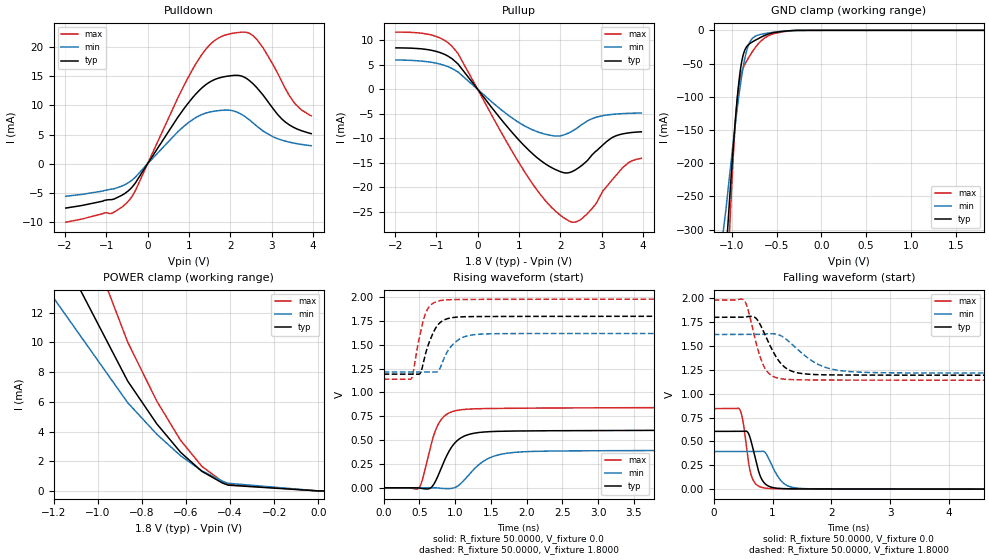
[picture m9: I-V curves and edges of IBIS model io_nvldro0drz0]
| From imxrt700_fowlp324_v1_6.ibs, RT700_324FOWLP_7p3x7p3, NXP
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[Model] io_nvldro0drz0
|   Model io_nvldro0drz0
| This model was characterised for following simulation conditions:
| External (pad) voltage:
|   - Typ: 1.8V,   - Min: 1.62V,   - Max: 1.98V
| Library cells for typ/min/max conditions are connected as defined below:
|  ipp_io - External Pad
|  ipp_do - Core Input
|  ipp_obe - Output Buffer Enable
|  config1v21v8 - gnde
|  drive0 - gnd
|  drive1 - gnd
|  gnd - gnd
|  gnde - gnde
|  ncgather - NC
|  vdd - vdd
|  vdde1v8 - vdde1v8
| All other pins connected to ground
Model_type I/O
Polarity   Non-Inverting
Enable   Active-Low
Vinl =   0.5400V
Vinh =   1.2600V
Vmeas =  0.9000V
Cref =   30.0000pF
Rref =   1.0000M
Vref =   1.8000V
C_comp   2.6144pF   2.5653pF   2.7096pF
|C_comp_pullup   1.3317pF   1.3902pF   1.2759pF
|C_comp_pulldown   0.0F   0.0F   0.0F
[Model Spec]
| variable   typ   min   max
Vinh   1.2600V   NA   NA
Vinl   0.5400V   NA   NA
Vref   1.8000V   1.8000V   1.8000V
Cref   30.0000pF   30.0000pF   30.0000pF
Rref   1.0000M   1.0000M   1.0000M
[Temperature Range]   25.0000   0.1250k   -40.0000
[Voltage Range]   1.8000V   1.6200V   1.9800V
[Pullup Reference]   1.8000V   1.6200V   1.9800V
[Pulldown Reference]   0.0V   0.0V   0.0V
[POWER Clamp Reference]   1.8000V   1.6200V   1.9800V
[GND Clamp Reference]   0.0V   0.0V   0.0V
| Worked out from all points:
|   slope of the pulldown table from 0 to 0.27 V, typ, clamps not added: 91.8 ohm
|   slope of the pullup table from 0 to 0.27 V, typ, clamps not added: 90.9 ohm
|   GND clamp passes 1 mA (typ) near -0.39 V on its own axis
|   POWER clamp passes 1 mA (typ) near -0.49 V on its own axis
|   rising waveform, R_fixture 50.0000, V_fixture 0.0: 20-80 % time 255ps typ, 362ps min, 198ps max; typ from 0 V to 0.605 V
|   rising waveform, R_fixture 50.0000, V_fixture 1.8000: 20-80 % time 173ps typ, 209ps min, 142ps max; typ from 1.19 V to 1.8 V
|   falling waveform, R_fixture 50.0000, V_fixture 0.0: 20-80 % time 159ps typ, 220ps min, 121ps max; typ from 0.605 V to 0 V
|   falling waveform, R_fixture 50.0000, V_fixture 1.8000: 20-80 % time 319ps typ, 521ps min, 225ps max; typ from 1.8 V to 1.19 V
[Pulldown]
|Voltage   I(typ)   I(min)   I(max)
-1.98V    -7.616mA   -5.589mA   -10.04mA
-876mV    -6.173mA   -4.375mA   -8.533mA
-468mV    -4.664mA   -3.281mA   -6.446mA
1.104V    11.45mA    7.63mA     16.37mA
1.464V    13.83mA    8.787mA    20.09mA
1.8V      14.84mA    9.158mA    21.85mA
2.232V    15.1mA     8.619mA    22.54mA
2.544V    13.77mA    7.047mA    22mA
2.796V    11.75mA    5.585mA    19.87mA
3.336V    7.128mA    3.861mA    12.86mA
3.624V    5.93mA     3.417mA    9.865mA
3.96V     5.157mA    3.077mA    8.199mA
[Pullup]
|Voltage   I(typ)   I(min)   I(max)
-1.98V    8.467mA    6.01mA     11.69mA
-1.104V   7.947mA    5.496mA    11.06mA
-624mV    6.265mA    4.273mA    8.816mA
-480mV    5.208mA    3.563mA    7.35mA
1.128V    -11.53mA   -7.445mA   -16.76mA
1.704V    -15.58mA   -9.295mA   -23.38mA
2.22V     -16.99mA   -8.831mA   -26.93mA
2.364V    -16.45mA   -8.142mA   -27.12mA
2.652V    -14.56mA   -6.463mA   -25.4mA
3.228V    -9.987mA   -5.14mA    -18.75mA
3.66V     -8.885mA   -4.9mA     -14.92mA
3.96V     -8.674mA   -4.832mA   -14.09mA
[GND_clamp]
|Voltage   I(typ)   I(min)   I(max)
-1.98V    -2.304A    -1.314A    -3.648A
-1.188V   -579.3mA   -402.9mA   -809.8mA
-1.068V   -345.9mA   -273.9mA   -436.6mA
-1.02V    -246.9mA   -214.1mA   -290.1mA
-972mV    -156.3mA   -155.7mA   -166mA
-924mV    -82.86mA   -102.6mA   -86.85mA
-864mV    -33.43mA   -49.36mA   -54.12mA
-816mV    -21.98mA   -23.37mA   -42.16mA
-744mV    -15.43mA   -9.445mA   -27.16mA
-588mV    -5.426mA   -3.899mA   -8.058mA
-312mV    -266.2uA   -304.2uA   -358.5uA
1.812V    32.97nA    19.92uA    18.44nA
[POWER_clamp]
|Voltage   I(typ)   I(min)   I(max)
-1.98V    42.17mA    31.68mA    56.98mA
-1.428V   23.53mA    17.8mA     32mA
-864mV    7.406mA    5.949mA    10.03mA
-732mV    4.524mA    3.821mA    6.055mA
-624mV    2.605mA    2.373mA    3.409mA
-528mV    1.324mA    1.357mA    1.664mA
-432mV    516uA      643.3uA    600.9uA
-408mV    387.6uA    513.5uA    443.1uA
0V        28.12nA    179.8nA    22.83nA
24mV      22.85nA    114.3nA    21.08nA
[Ramp]
| variable   typ   min   max
dV/dt_r  0.3630/0.2552n   0.2364/0.3617n   0.5061/0.1976n
dV/dt_f  0.3644/0.3188n   0.2429/0.5209n   0.5041/0.2247n
R_load = 50.0000
[Rising Waveform]
R_fixture= 50.0000
V_fixture= 0.0
V_fixture_min= 0.0
V_fixture_max= 0.0
|time   V(typ)   V(min)   V(max)
0s        390.4nV    3.833uV    891.1nV
484.1ps   -1.093mV   3.418uV    -8.772mV
542.3ps   -7.742mV   4.279uV    85.28mV
665.9ps   3.522mV    -8.561uV   460.7mV
813.7ps   220.3mV    -6.258mV   724.1mV
1.042ns   503.5mV    21.94mV    813.8mV
1.394ns   584.4mV    277.3mV    830.8mV
1.888ns   595.8mV    374.6mV    834.9mV
3.742ns   602mV      390.5mV    840.6mV
60ns      605mV      394mV      843.5mV
[Rising Waveform]
R_fixture= 50.0000
V_fixture= 1.8000
V_fixture_min= 1.6200
V_fixture_max= 1.9800
|time   V(typ)   V(min)   V(max)
0s        1.193V     1.215V     1.14V
385.6ps   1.193V     1.215V     1.142V
514.1ps   1.204V     1.215V     1.626V
614ps     1.478V     1.215V     1.873V
779.9ps   1.726V     1.241V     1.962V
896.6ps   1.775V     1.436V     1.972V
1.029ns   1.791V     1.544V     1.975V
1.29ns    1.797V     1.608V     1.977V
2.062ns   1.798V     1.618V     1.978V
60ns      1.8V       1.62V      1.98V
[Falling Waveform]
R_fixture= 50.0000
V_fixture= 0.0
V_fixture_min= 0.0
V_fixture_max= 0.0
|time   V(typ)   V(min)   V(max)
0s        605mV      394mV      843.5mV
437.5ps   605mV      394mV      838mV
495.5ps   604.7mV    394mV      714.8mV
574.9ps   597.6mV    394mV      352.9mV
660.6ps   439.3mV    394mV      106.4mV
813.1ps   106.5mV    396.2mV    18.68mV
1.031ns   13.6mV     194.9mV    5.256mV
1.287ns   3.953mV    27.56mV    3.692mV
1.856ns   2.25mV     2.345mV    2.708mV
60ns      713.8nV    7.047uV    916.2nV
[Falling Waveform]
R_fixture= 50.0000
V_fixture= 1.8000
V_fixture_min= 1.6200
V_fixture_max= 1.9800
|time   V(typ)   V(min)   V(max)
0s        1.8V       1.62V      1.98V
511.6ps   1.8V       1.62V      1.98V
581.1ps   1.808V     1.62V      1.883V
715.5ps   1.791V     1.62V      1.542V
883.7ps   1.6V       1.626V     1.252V
1.137ns   1.319V     1.609V     1.157V
1.408ns   1.22V      1.473V     1.145V
1.992ns   1.196V     1.259V     1.143V
3.052ns   1.194V     1.218V     1.141V
60ns      1.193V     1.215V     1.14V
